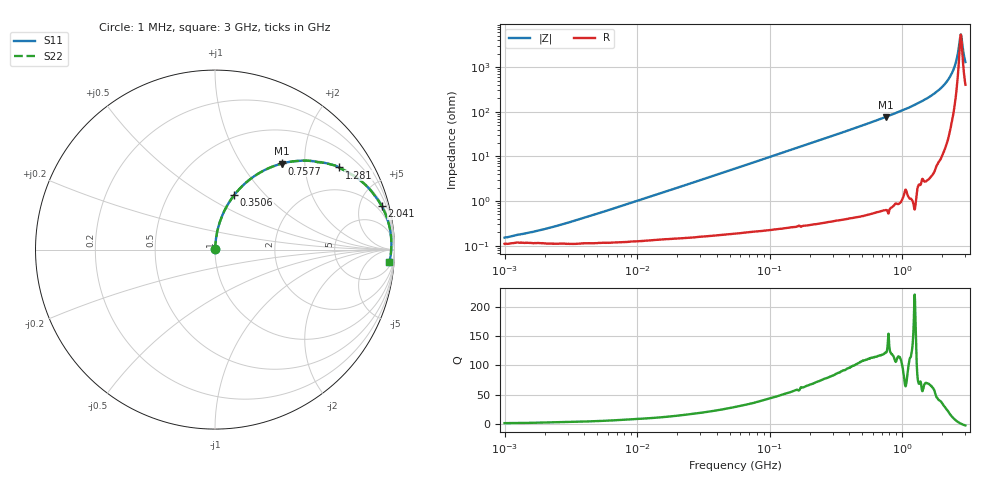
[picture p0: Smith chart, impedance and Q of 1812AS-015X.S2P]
!s-Parameter Generated by FASTRON Sdn. Bhd.
!FASTRON P/N : 1812AS-015X
!Keysight Technologies,E4991B,MY54100416,A.01.15
!Date created: Fri Oct 13 13:37:43 2023
!Version  : Rev00 Fri Oct 13 13:37:43 2023
!Data & Calibration Information:
!Freq	S11	S21	S12	S22
!PortZ  Port1:50+j0  Port2:50+j0
!When reading, reference impedance value at option line is always used.
! Remarks : This data is being provided solely for informational purposes.
# Hz S dB R 50
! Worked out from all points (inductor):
!   1601 points, 1 MHz to 3 GHz, reference 50 ohm
!   read as one part in series: L = 16.2 nH near 3.225 MHz
!   highest Q = 122 at 753.9 MHz (marker M1), where L = 16.2 nH
!   self-resonance near 2.769 GHz
!   S11 on the Smith chart (normalised r, x): 1 MHz: 1.00, +0.00; 350.6 MHz: 1.01, +0.68; 757.7 MHz: 1.01, +1.54; 1.281 GHz: 1.03, +3.00; 2.041 GHz: 1.24, +7.60; 3 GHz: 9, -25
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1000000  -56.42 43.2  -0.01 -0.1  -0.01 -0.1  -56.42 43.2
2045350  -52.45 62.0  -0.01 -0.1  -0.01 -0.1  -52.45 62.0
3804036  -47.88 73.7  -0.01 -0.2  -0.01 -0.2  -47.88 73.7
1.447069e7  -36.85 83.8  -0.01 -0.8  -0.01 -0.8  -36.85 83.8
5.477226e7  -25.51 85.0  -0.03 -3.0  -0.03 -3.0  -25.51 85.0
2.083556e8  -14.13 77.8  -0.20 -11.3  -0.20 -11.3  -14.13 77.8
3.50605e8  -9.87 70.6  -0.51 -18.7  -0.51 -18.7  -9.87 70.6
5.205962e8  -6.85 62.4  -1.05 -27.0  -1.05 -27.0  -6.85 62.4
7.539071e8  -4.35 52.2  -2.04 -37.3  -2.04 -37.3  -4.35 52.2
7.576891e8  -4.32 52.1  -2.06 -37.5  -2.06 -37.5  -4.32 52.1
7.925923e8  -4.03 50.7  -2.23 -38.9  -2.23 -38.9  -4.03 50.7
1.281378e9  -1.63 33.5  -5.16 -56.0  -5.16 -56.0  -1.63 33.5
1.662201e9  -0.80 23.3  -8.04 -65.8  -8.04 -65.8  -0.80 23.3
2.040726e9  -0.36 14.6  -11.96 -73.6  -11.96 -73.6  -0.36 14.6
2.255531e9  -0.22 10.1  -15.14 -76.9  -15.14 -76.9  -0.22 10.1
2.431346e9  -0.16 6.5  -18.84 -77.6  -18.84 -77.6  -0.16 6.5
2.543347e9  -0.14 4.3  -22.30 -75.5  -22.30 -75.5  -0.14 4.3
2.687267e9  -0.15 1.6  -29.83 -58.1  -29.83 -58.1  -0.15 1.6
2.741597e9  -0.15 0.6  -33.88 -28.9  -33.88 -28.9  -0.15 0.6
2.825159e9  -0.17 -1.0  -31.88 40.3  -31.88 40.3  -0.17 -1.0
2.940549e9  -0.21 -3.1  -24.72 64.7  -24.72 64.7  -0.21 -3.1
3e9  -0.23 -4.1  -22.50 67.9  -22.50 67.9  -0.23 -4.1
